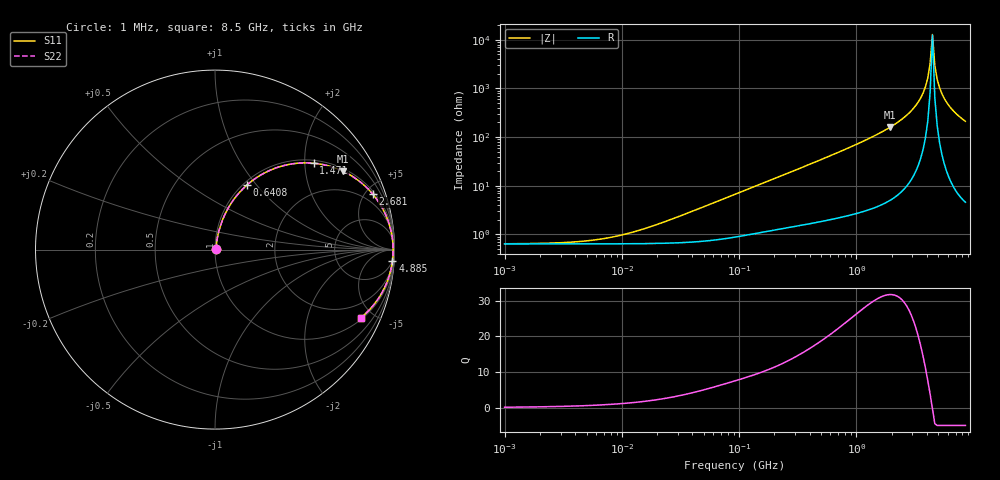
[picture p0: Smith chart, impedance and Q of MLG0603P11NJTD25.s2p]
! S-Parameter Data Generated by TDK Corporation
! Copyright(C) 2025 TDK Corporation.
! All Rights Reserved.
! TDK P/N: MLG0603P11NJTD25 (SMD / SMT Inductor (Coil))
! Property: L=11nH at 500MHz
! Size(LxWxT): 0.6x0.3x0.3mm
! Model Type: s2p (Touchstone File Format Version 1.0)
! Frequency: DC=Yes Start=1MHz Stop=8500MHz 198points Log-sweep
! Model Generated on Feb. 6, 2025
! Terms and conditions regarding TDK Simulation Models:
! 1)This simulation model is being provided solely for informational
!  purposes. Please refer to the specifications of the products in
!  terms of detailed characteristics of such products.
! 2)In no event shall TDK Corporation of any of its subsidiaries be
!  liable for any loss or damage arising, directly or indirectly,
!  from any information contained in this simulation model, including,
!  but not limited to loss or damages arising from any inaccuracies,
!  omissions or errors in connection with such information.
! 3)Any and all copyrights on this simulation model are owned by
!  TDK Corporation.  Duplication or redistribution of this simulation
!  model without prior written permission from TDK Corporation
!  is prohibited.
! 4)This simulation model is subject to any modification or change
!  without any prior notice.
! 5)Neither TDK Corporation nor any of its subsidiaries shall make any
!  warranty, express or implied, including but not limited to the
!  correctness, implied warranties of merchantability and fitness for
!  a particular purpose with respect to this simulation models.
! 6)The use of this simulation model shall be deemed to have consented
!  to the terms and conditions hereof.
! Port Assignments:
!  1 ---@@@--- 2
! Applicable Conditions:
!  Temperature = 25 degC
!  DC Bias Current = 0 A
!  Small Signal Operation
# Hz S MA R 50
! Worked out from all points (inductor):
!   197 points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, 1 MHz to 8.5 GHz, reference 50 ohm
!   read as one part in series: L = 11.7 nH near 27.76 MHz
!   highest Q = 31.7 at 1.94 GHz (marker M1), where L = 13.1 nH
!   self-resonance near 4.253 GHz
!   S11 on the Smith chart (normalised r, x): 1 MHz: 1.01, +0.00; 640.8 MHz: 1.04, +0.89; 1.471 GHz: 1.07, +2.21; 2.681 GHz: 1.20, +5.62; 4.885 GHz: 4, -31; 8.5 GHz: 1.09, -4.23
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1000000  0.006402 6.5  0.9936 -0.0  0.9936 -0.0  0.006402 6.5
4587603  0.007198 27.6  0.9936 -0.2  0.9936 -0.2  0.007198 27.6
9601846  0.009498 47.3  0.9936 -0.4  0.9936 -0.4  0.009498 47.3
2.10461e7  0.0167 66.1  0.9934 -0.9  0.9934 -0.9  0.0167 66.1
9.219544e7  0.06629 78.7  0.9891 -3.8  0.9891 -3.8  0.06629 78.7
4.229561e8  0.2767 70.6  0.945 -16.0  0.945 -16.0  0.2767 70.6
6.408078e8  0.3995 63.8  0.8982 -23.5  0.8982 -23.5  0.3995 63.8
9.708683e8  0.5567 54.0  0.8096 -33.8  0.8096 -33.8  0.5567 54.0
1.470933e9  0.7304 41.2  0.6594 -46.9  0.6594 -46.9  0.7304 41.2
1.940355e9  0.8367 31.5  0.522 -56.7  0.522 -56.7  0.8367 31.5
2.680511e9  0.9319 19.4  0.3317 -68.6  0.3317 -68.6  0.9319 19.4
3.37643e9  0.974 10.5  0.1831 -76.6  0.1831 -76.6  0.974 10.5
3.877948e9  0.9877 5.2  0.09135 -79.7  0.09135 -79.7  0.9877 5.2
4.061159e9  0.9903 3.4  0.06061 -79.1  0.06061 -79.1  0.9903 3.4
4.253027e9  0.9919 1.7  0.0301 -73.6  0.0301 -73.6  0.9919 1.7
4.453958e9  0.9925 -0.1  0.007715 14.3  0.007715 14.3  0.9925 -0.1
4.664383e9  0.9921 -1.9  0.03377 75.6  0.03377 75.6  0.9921 -1.9
4.884749e9  0.9907 -3.7  0.06442 79.9  0.06442 79.9  0.9907 -3.7
5.357206e9  0.9849 -7.2  0.1262 79.5  0.1262 79.5  0.9849 -7.2
5.87536e9  0.9751 -10.8  0.1877 77.0  0.1877 77.0  0.9751 -10.8
6.748056e9  0.9528 -16.2  0.2786 72.3  0.2786 72.3  0.9528 -16.2
8.5e9  0.8966 -25.1  0.4237 63.7  0.4237 63.7  0.8966 -25.1
